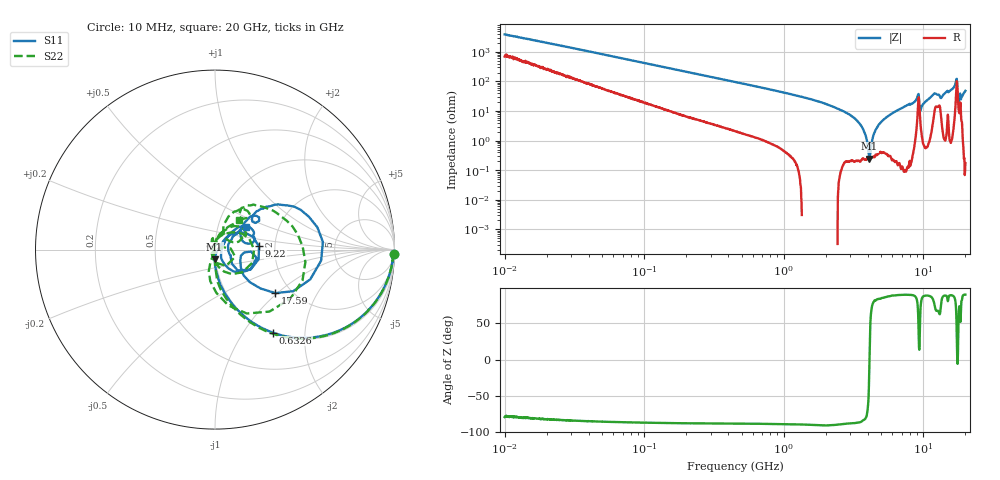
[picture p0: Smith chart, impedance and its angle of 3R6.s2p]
!Keysight Technologies,P5008B,MY61100088,A.16.20.02
!Date: Monday, October 30, 2023 16:39:00
!Correction: S11(C  2-Port  )
!S21(C  2-Port  )
!S12(C  2-Port  )
!S22(C  2-Port  )
!S2P File: Measurements: S11, S21, S12, S22:Log Frequency Sweep
# Hz S  dB  R 50
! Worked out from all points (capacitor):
!   1601 points, 10 MHz to 20 GHz, reference 50 ohm
!   read as one part in series: C = 4.07 pF near 10.39 MHz
!   lowest |Z| = 243 mohm at 4.112 GHz (marker M1)
!   series resonance near 4.107 GHz, so ESL is about 370 pH
!   S11 on the Smith chart (normalised r, x): 10 MHz: 14, -76; 632.6 MHz: 1.01, -1.37; 9.22 GHz: 1.65, +0.07; 17.59 GHz: 1.66, -0.97; 20 GHz: 1.36, +0.36
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1e7  -0.04 -1.5  -31.84 78.2  -31.85 78.2  -0.04 -1.5
3.555162e7  -0.09 -4.9  -21.45 80.3  -21.46 80.3  -0.09 -4.9
1.263918e8  -0.46 -16.3  -11.06 71.3  -11.06 71.3  -0.46 -16.5
4.472136e8  -3.23 -45.5  -2.98 43.0  -2.99 43.0  -3.23 -46.0
6.325932e8  -5.00 -55.2  -1.76 33.4  -1.77 33.4  -5.00 -56.0
1.589917e9  -11.84 -76.9  -0.28 12.7  -0.29 12.7  -11.83 -79.0
4.111527e9  -25.16 -92.5  -0.03 -3.2  -0.03 -3.2  -25.30 -88.5
5.067356e9  -31.72 -81.8  -0.02 -6.7  -0.02 -6.7  -32.15 -86.0
5.652411e9  -35.93 -54.9  -0.01 -8.7  -0.01 -8.7  -39.14 -105.5
6.069891e9  -36.72 -10.5  -0.00 -10.1  -0.00 -10.1  -44.62 172.0
7.202016e9  -27.68 30.1  -0.00 -13.9  -0.01 -14.0  -28.26 117.3
8.344716e9  -25.99 41.2  -0.02 -18.4  -0.02 -18.4  -26.28 91.9
9.220141e9  -12.18 4.4  -2.02 -23.8  -2.03 -23.9  -13.23 0.2
9.761022e9  -27.34 -38.2  -0.09 -18.0  -0.09 -18.0  -34.99 -124.9
9.995649e9  -28.98 -2.4  -0.03 -19.8  -0.04 -19.9  -36.83 125.3
1.185999e10  -13.44 38.1  -0.66 -31.0  -0.67 -31.1  -14.54 43.3
1.335558e10  -15.79 15.9  -0.66 -24.6  -0.66 -24.7  -20.97 52.6
1.599787e10  -9.32 41.6  -0.64 -43.1  -0.64 -43.1  -9.65 49.6
1.685609e10  -6.46 31.1  -1.85 -54.1  -1.85 -54.2  -7.33 22.1
1.75924e10  -7.64 -35.7  -3.45 -17.1  -3.45 -17.2  -9.90 -76.5
1.862442e10  -18.12 -40.1  -0.69 -31.6  -0.69 -31.7  -30.48 -126.7
2e10  -13.45 35.9  -0.25 -46.8  -0.25 -46.9  -13.54 51.0
